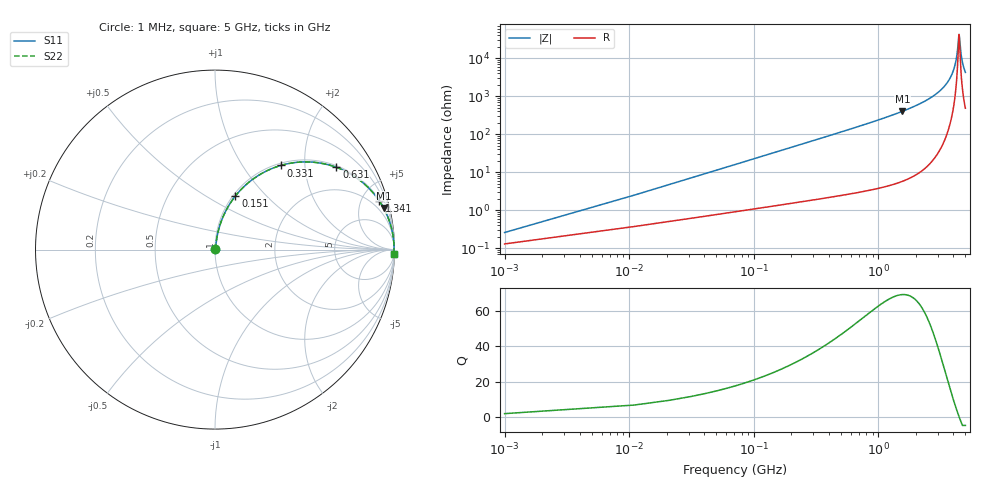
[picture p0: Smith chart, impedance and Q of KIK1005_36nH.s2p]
!version-3
!date-01.2023
!Series
# MHz S RI R 50
!Freq ReS11 ImS11 ReS21 ImS21 ReS12 ImS12 ReS22 ImS22
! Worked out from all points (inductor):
!   501 points, 1 MHz to 5 GHz, reference 50 ohm
!   read as one part in series: L = 36 nH near 21 MHz
!   highest Q = 69.5 at 1.561 GHz (marker M1), where L = 41.1 nH
!   self-resonance near 4.441 GHz
!   S11 on the Smith chart (normalised r, x): 1 MHz: 1.00, +0.00; 151 MHz: 1.03, +0.68; 331 MHz: 1.04, +1.51; 631 MHz: 1.06, +2.91; 1.341 GHz: 1.10, +6.67; 5 GHz: 11, -85
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1  0.00131 0.00226  0.9987 -0.00226  0.9987 -0.00226  0.00131 0.00226
31  0.0109 0.0689  0.9891 -0.0689  0.9891 -0.0689  0.0109 0.0689
41  0.0153 0.0907  0.9847 -0.0907  0.9847 -0.0907  0.0153 0.0907
81  0.0413 0.174  0.9587 -0.174  0.9587 -0.174  0.0413 0.174
151  0.114 0.299  0.886 -0.299  0.886 -0.299  0.114 0.299
331  0.3653 0.4686  0.6347 -0.4686  0.6347 -0.4686  0.3653 0.4686
631  0.6766 0.4583  0.3234 -0.4583  0.3234 -0.4583  0.6766 0.4583
841  0.7916 0.3977  0.2084 -0.3977  0.2084 -0.3977  0.7916 0.3977
1341  0.9143 0.2728  0.0857 -0.2728  0.0857 -0.2728  0.9143 0.2728
1561  0.939 0.2323  0.061 -0.2323  0.061 -0.2323  0.939 0.2323
1671  0.9481 0.2147  0.0519 -0.2147  0.0519 -0.2147  0.9481 0.2147
2501  0.9835 0.1186  0.0165 -0.1186  0.0165 -0.1186  0.9835 0.1186
3341  0.9947 0.0572  0.00529 -0.0572  0.00529 -0.0572  0.9947 0.0572
3851  0.9971 0.0286  0.00292 -0.0286  0.00292 -0.0286  0.9971 0.0286
4171  0.9976 0.0127  0.00238 -0.0127  0.00238 -0.0127  0.9976 0.0127
4291  0.9977 0.00706  0.00233 -0.00706  0.00233 -0.00706  0.9977 0.00706
4421  0.9977 0.00115  0.00234 -0.00115  0.00234 -0.00115  0.9977 0.00115
4451  0.9976 -0.000184  0.00235 0.000184  0.00235 0.000184  0.9976 -0.000184
4581  0.9975 -0.00588  0.00246 0.00588  0.00246 0.00588  0.9975 -0.00588
4671  0.9974 -0.00973  0.00257 0.00973  0.00257 0.00973  0.9974 -0.00973
4821  0.9972 -0.016  0.00282 0.016  0.00282 0.016  0.9972 -0.016
5000  0.9968 -0.0232  0.00322 0.0232  0.00322 0.0232  0.9968 -0.0232
